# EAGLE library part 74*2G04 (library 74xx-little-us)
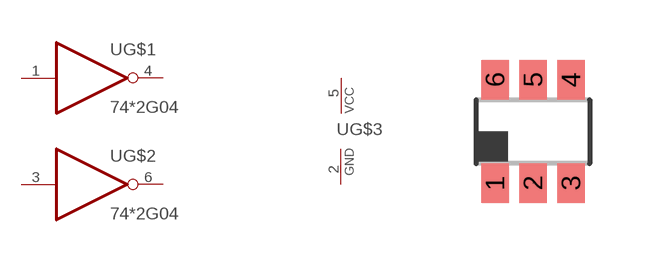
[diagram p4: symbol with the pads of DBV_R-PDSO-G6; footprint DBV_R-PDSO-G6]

Designator prefix -; gates G$1=7404 G$2=7404 G$3=PWRN

## 742G04-SO6  [DBV_R-PDSO-G6]
1  G$1:I  in
2  G$3:GND  pwr
3  G$2:I  in
4  G$1:O  out
5  G$3:VCC  pwr
6  G$2:O  out

## Footprint DBV_R-PDSO-G6 (pad centres in mm)
DBV (R-PDSO-G6) PLASTIC SMALL-OUTLINE PACKAGE SOT (SOT-23) - DBV Source: http://focus.ti.com/lit/ds/symlink/sn74lvc1g3157.
smd 0.69 x 0.99: 1 -0.95,-1.29; 2 0,-1.29; 3 0.95,-1.29; 4 0.95,1.3; 5 0,1.3; 6 -0.95,1.3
